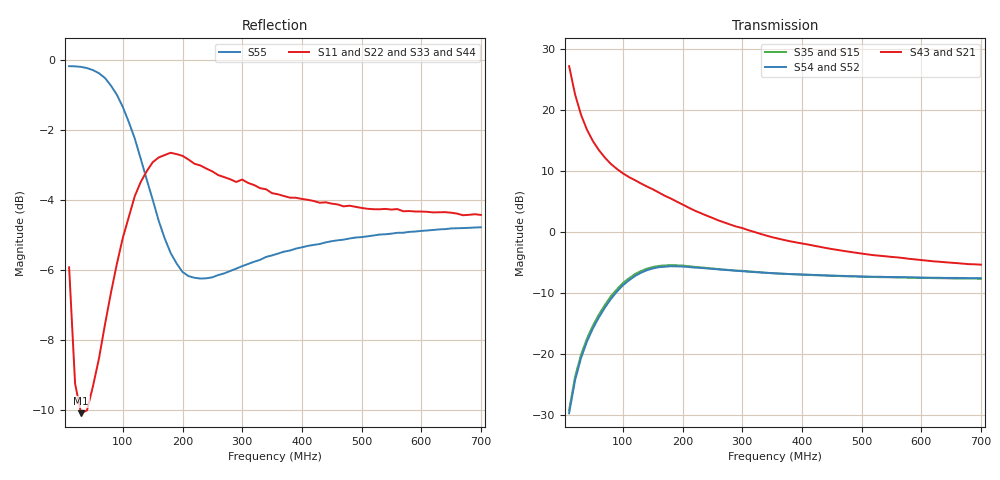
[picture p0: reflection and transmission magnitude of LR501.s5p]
!  POLYFET RF DEVICES
!  LR501 (Each Side)
!  S PARAMETERS
!  VDS=28V, IDQ=400mA
! Date: Thu Mar 13 09:54:24 2003
!AWR Design Environment (2053) Wed Feb 04 15:27:10 2004
!freq-unit  param-type  data-format  keyword  impedance-ohms
# MHz  S  MA  R  50
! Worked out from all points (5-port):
!   70 points, 10 MHz to 700 MHz, reference 50 ohm
!   strongest paths, dB at 10 MHz, 180 MHz, 360 MHz, 530 MHz, 700 MHz:
!     S43: 27.2, 5.5, -1.1, -3.9, -5.3
!     S21: 27.2, 5.5, -1.1, -3.9, -5.3
!     S54: -29.7, -5.6, -6.8, -7.3, -7.5
!     S52: -29.7, -5.6, -6.8, -7.3, -7.5
!     S35: -29.2, -5.4, -6.8, -7.4, -7.6
!     S15: -29.2, -5.4, -6.8, -7.4, -7.6
!   lowest |S11| = -10.1 dB at 30 MHz (marker M1), VSWR 1.91, Z = 52 - j33.5 ohm
!   |S11| at or under -10 dB: 28.83 MHz to 40.21 MHz (11.38 MHz wide, 33 % of centre)
